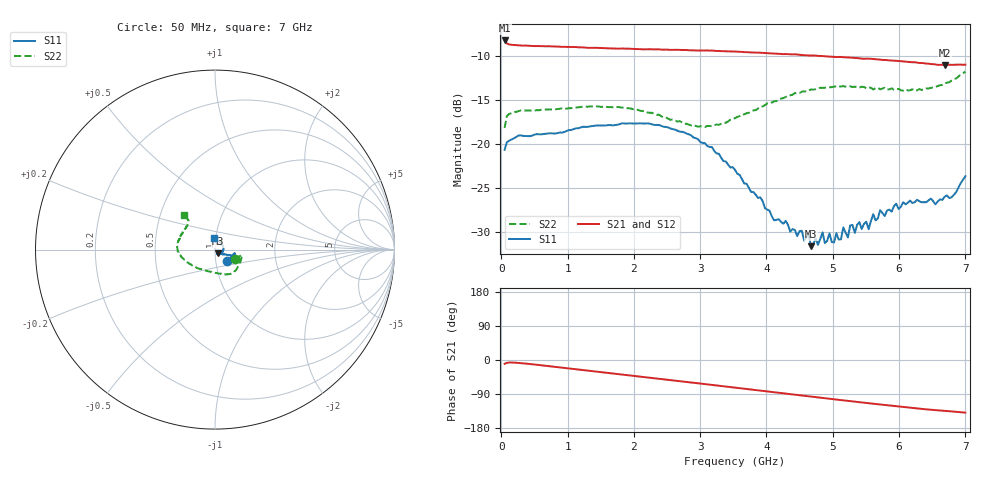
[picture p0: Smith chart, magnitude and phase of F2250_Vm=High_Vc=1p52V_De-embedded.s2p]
! Integrated Device Technology
! Corporate Headquarters
! 6024 Silver Creek Valley Road
! San Jose, CA 95138  USA
! Phone:  1-408-284-8200
! Toll Free:  1-800-223-1366
! Webpage:  http://www.idt.com/
! Timing and RF Division
! 515 Groton Road, Suite 102
! Westford, MA 01886-6024
! Device:  F2250
! Description: Voltage Variable RF Attenuator
! Frequency:  50.0 -  6000.00 MHz
! Package:  3x3 mm Thin QFN Plastic Package: 16 pin
! Ports:  2 RF, 3 DC
!  Pin  1  = GND
!  Pin  2  = NC
!  Pin  3  = RF1  = Port 1
!  Pin  4  = NC
!  Pin  5  = GND
!  Pin  6  = GND
!  Pin  7  = GND
!  Pin  8  = GND
!  Pin  9  = NC
!  Pin 10  = RF2  = Port 2
!  Pin 11  = NC
!  Pin 12  = GND
!  Pin 13  = GND
!  Pin 14  = VCNTRL
!  Pin 15  = VDD
!  Pin 16  = VMODE
! Vcntrl:  1.520 Volts
! Vmode:  +3.300 Volts
! Vdd:  +3.30  Volts
! Current:  1.327 mA
! Data:  The device was measured on a the F2250 evaluation board which has
!  individual transmission lines to the RF pins.  Data was collected
!  using a calibrated network analyzer.  The evaluation board was
!  de-embedded using a TRL calibration technique.
!  The reference plane is the edge of the package pin.
! Misc:  SN 10
!  Action Tracker AT0258
! Date Measured:  2014-11-26
! Date:  2015-10-15  MJV
! Note:
!  Integrated Device Technology supplies this data as a sample of measured
!  data at the package pin for this product.  Your particular data for this
!  product may vary.
!  Data was taken at 25 degrees C.
!  Integrated Device Technology reserves the right to change this data at anytime.
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# GHz S dB R 50
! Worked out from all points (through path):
!   201 points, 50 MHz to 7 GHz, reference 50 ohm
!   highest |S21| = -8.25 dB at 50 MHz (marker M1); lowest = -11.0 dB at 6.687 GHz (marker M2)
!   group delay of S21, straight-line fit = 55.5 ps
!   lowest |S11| = -31.6 dB at 4.672 GHz (marker M3), VSWR 1.05, Z = 51.5 - j2.19 ohm
!   |S11| at or under -10 dB: start of sweep to end of sweep
!   |S22| runs from -18.2 to -11.8 dB; largest |S21 - S12| = 0.0017
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0.05  -20.64 -42.6  -8.25 -10.0  -8.26 -10.0  -18.17 -26.2
0.189  -19.34 -12.0  -8.77 -6.8  -8.77 -6.8  -16.40 -11.4
1.2315  -18.03 -21.9  -9.04 -26.5  -9.05 -26.5  -15.74 -42.3
2.37825  -17.83 -21.3  -9.25 -49.3  -9.27 -49.4  -16.66 -70.6
2.969  -19.45 -18.6  -9.40 -61.5  -9.38 -61.5  -18.04 -98.0
3.525  -22.91 -23.5  -9.51 -73.1  -9.52 -73.1  -17.06 -131.9
4.11575  -28.63 -40.9  -9.74 -85.3  -9.71 -85.3  -15.14 -158.6
4.637  -30.31 -53.2  -9.95 -95.9  -9.94 -96.0  -13.90 -174.5
4.67175  -31.56 -53.6  -9.95 -96.7  -9.94 -96.7  -13.81 -174.8
4.7065  -31.31 -62.5  -9.95 -97.4  -9.95 -97.4  -13.83 -175.5
4.8455  -30.00 -58.8  -10.02 -100.1  -10.01 -100.2  -13.62 -178.5
4.88025  -31.20 -55.5  -10.05 -100.8  -10.04 -100.9  -13.61 -179.8
5.1235  -30.79 -59.3  -10.12 -105.8  -10.13 -105.8  -13.46 174.4
5.15825  -29.44 -54.7  -10.15 -106.4  -10.15 -106.5  -13.44 173.9
5.22775  -30.58 -51.7  -10.17 -107.9  -10.16 -107.9  -13.42 172.1
5.2625  -29.22 -50.1  -10.19 -108.5  -10.19 -108.5  -13.44 171.7
5.4015  -28.84 -35.8  -10.28 -111.3  -10.25 -111.4  -13.59 167.5
5.5405  -29.64 -33.1  -10.31 -114.1  -10.29 -114.2  -13.56 164.0
5.61  -27.93 -30.4  -10.35 -115.4  -10.35 -115.5  -13.80 162.7
5.85325  -27.42 -18.4  -10.51 -120.1  -10.52 -120.2  -13.79 155.4
6.68725  -25.96 51.2  -11.05 -134.2  -11.04 -134.4  -13.13 132.1
7  -23.63 97.2  -11.00 -138.9  -11.00 -139.1  -11.77 131.6
